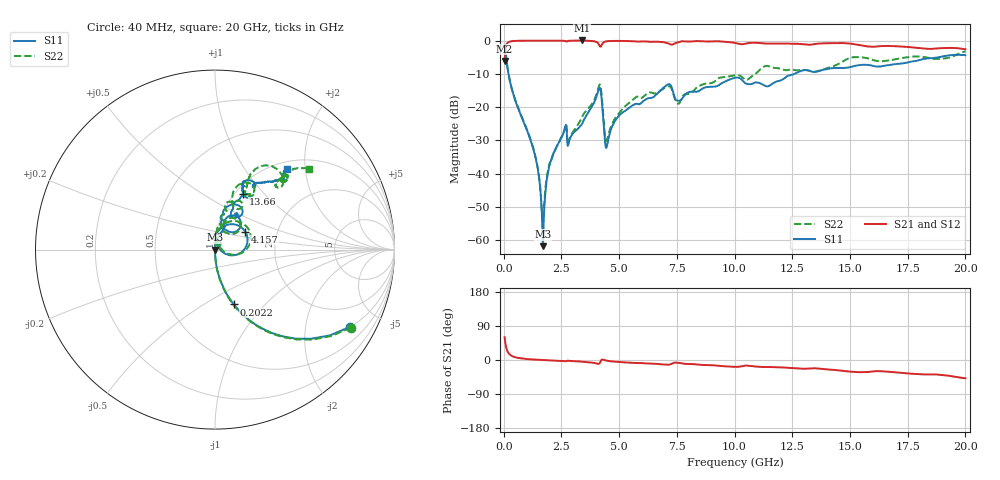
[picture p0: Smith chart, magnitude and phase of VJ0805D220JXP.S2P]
! VJ0805D220JXP
! DATE 10/29/2021  12:18
! CAPACITORS MOUNTED IN SERIES ON 25 MIL THICK MICROSTRIP SUBSTRATE
# GHz  S  MA  R  50.00
!  FREQ  S11M  S11A  S21M  S21A  S12M  S12A  S22M  S22A
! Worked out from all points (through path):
!   1601 points, 40 MHz to 20 GHz, reference 50 ohm
!   highest |S21| = 0.05 dB at 3.396 GHz (marker M1); lowest = -6.2 dB at 40 MHz (marker M2)
!   group delay of S21, straight-line fit = 6.68 ps
!   lowest |S11| = -61.8 dB at 1.699 GHz (marker M3), VSWR 1.00, Z = 50.1 - j0.00239 ohm
!   |S11| at or under -10 dB: 207.1 MHz to 12.59 GHz (12.38 GHz wide, 194 % of centre)
!   |S22| runs from -56.0 to -1.2 dB; largest |S21 - S12| = 0.008
!   S11 on the Smith chart (normalised r, x): 40 MHz: 1.01, -3.50; 202.2 MHz: 1.00, -0.68; 4.157 GHz: 1.37, +0.29; 13.66 GHz: 1.08, +0.77; 20 GHz: 1.14, +1.61
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0.04  0.8673 -29.7  0.4923 60.0  0.494 60.2  0.8731 -30.0
0.202175  0.3232 -71.0  0.946 18.9  0.9457 18.8  0.3271 -71.4
1.3374  0.02005 -88.8  0.9988 0.9  0.9987 0.9  0.02082 -86.0
1.699175  0.0008101 -1.7  0.9983 -0.3  0.9983 -0.4  0.001583 9.9
1.9362  0.01098 79.2  0.9975 -1.0  0.9978 -1.1  0.01199 80.3
2.198175  0.02162 89.1  0.999 -1.7  0.9987 -1.7  0.02164 81.5
2.622325  0.04359 81.3  0.9948 -3.0  0.996 -3.2  0.04472 82.4
2.846875  0.0319 80.6  0.9957 -2.4  0.9966 -2.5  0.03279 83.8
3.370825  0.05435 90.3  1.006 -4.3  1.006 -4.4  0.06791 95.6
3.395775  0.05578 91.3  1.006 -4.4  1.006 -4.5  0.07083 95.3
4.15675  0.1959 30.9  0.8338 -8.6  0.835 -8.7  0.219 34.4
4.468625  0.02552 43.9  0.9783 -1.9  0.9789 -2.0  0.03207 43.7
5.042475  0.07703 74.7  0.9907 -5.4  0.9902 -5.5  0.08471 84.7
6.70165  0.1664 71.7  0.9626 -10.6  0.9631 -10.7  0.1693 70.5
7.163225  0.221 55.4  0.8975 -12.3  0.897 -12.4  0.2063 53.3
7.562425  0.1252 60.9  0.9467 -7.2  0.9466 -7.4  0.1123 57.9
10.02  0.2752 65.0  0.9225 -18.1  0.9228 -18.2  0.3015 65.0
11.42967  0.2053 61.4  0.903 -18.5  0.9024 -18.6  0.4165 60.0
13.35083  0.3417 57.5  0.8748 -21.8  0.8755 -22.1  0.3427 57.4
13.6627  0.3487 63.6  0.9046 -22.7  0.9047 -22.9  0.3536 61.7
16.68165  0.4283 58.7  0.8308 -31.2  0.8317 -31.6  0.5027 47.3
20  0.603 48.1  0.7412 -48.3  0.741 -48.7  0.692 40.7
